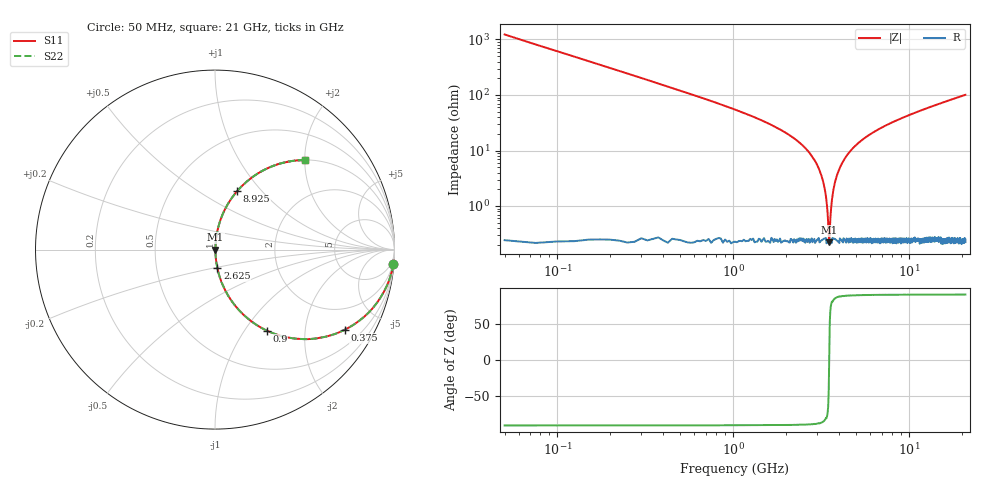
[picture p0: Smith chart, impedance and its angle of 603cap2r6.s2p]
! AVX Thin Film Operation		Date: November 2004
! Description: Accu-P® Series, Thin Film, SMD, RF Capacitor
! Part Number: 06035J2R6ABT
! 50 MHz  -  10.05 GHz
! Serial Measurements
# MHZ S MA R 50
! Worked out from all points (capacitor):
!   839 points, 50 MHz to 21 GHz, reference 50 ohm
!   read as one part in series: C = 2.6 pF near 150 MHz
!   lowest |Z| = 224 mohm at 3.525 GHz (marker M1)
!   series resonance near 3.521 GHz, so ESL is about 790 pH
!   S11 on the Smith chart (normalised r, x): 50 MHz: 1, -24; 375 MHz: 1.01, -3.23; 900 MHz: 1.00, -1.27; 2.625 GHz: 1.00, -0.21; 8.925 GHz: 1.00, +0.74; 21 GHz: 1.00, +2.02
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50  0.997 -4.7  0.081 85.3  0.081 85.3  0.997 -4.7
225  0.938 -20.3  0.346 69.7  0.346 69.7  0.938 -20.3
375  0.849 -31.8  0.526 58.2  0.526 58.2  0.849 -31.8
900  0.536 -57.4  0.842 32.4  0.842 32.4  0.536 -57.4
1550  0.303 -71.9  0.951 17.6  0.951 17.6  0.303 -71.9
2625  0.103 -82.8  0.992 5.9  0.992 5.9  0.103 -82.8
3200  0.033 -84.0  0.997 1.9  0.997 1.9  0.033 -84.0
3325  0.02 -82.0  0.997 1.1  0.997 1.1  0.02 -82.0
3450  0.007464 -70.8  0.998 0.4  0.998 0.4  0.007464 -70.8
3525  0.002431 9.3  0.998 -0.0  0.998 -0.0  0.002431 9.3
3550  0.003721 49.7  0.998 -0.2  0.998 -0.2  0.003721 49.7
3600  0.008061 72.2  0.998 -0.4  0.998 -0.4  0.008061 72.2
3700  0.017 81.1  0.997 -1.0  0.997 -1.0  0.017 81.1
3825  0.029 83.6  0.997 -1.6  0.997 -1.6  0.029 83.6
4350  0.074 83.9  0.995 -4.2  0.995 -4.2  0.074 83.9
5350  0.148 80.6  0.987 -8.5  0.987 -8.5  0.148 80.6
7050  0.252 74.9  0.965 -14.6  0.965 -14.6  0.252 74.9
8925  0.348 69.3  0.935 -20.4  0.935 -20.4  0.348 69.3
10525  0.418 65.0  0.906 -24.7  0.906 -24.7  0.418 65.0
14025  0.543 56.9  0.837 -32.9  0.837 -32.9  0.543 56.9
17525  0.638 50.2  0.768 -39.6  0.768 -39.6  0.638 50.2
21000  0.709 44.7  0.704 -45.2  0.704 -45.2  0.709 44.7
